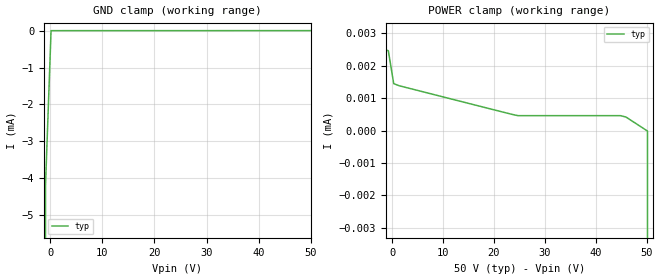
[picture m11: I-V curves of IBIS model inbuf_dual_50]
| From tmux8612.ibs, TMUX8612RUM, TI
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| inbuf_dual_50
[Model]   inbuf_dual_50
Model_type   Input
Vinl = 0.8
Vinh = 1.3
|   typ   min   max
C_comp   1.008417e-12   NA   NA
[Voltage Range]   50   NA   NA
[Temperature Range]   27   NA   NA
[Power Clamp Reference]   50   NA   NA
[GND Clamp Reference]   0   NA   NA
[GND Clamp]
|   Voltage   I(typ)   I(min)   I(max)
-55V      -12.6A     NA         NA
-1.97V    -208.8mA   NA         NA
-909.1mV  -4.166mA   NA         NA
151.5mV   15.32nA    NA         NA
50V       2.185uA    NA         NA
[POWER Clamp]
|   Voltage   I(typ)   I(min)   I(max)
-5V       5.025uA    NA         NA
-3.939V   2.591uA    NA         NA
-757.6mV  2.464uA    NA         NA
303mV     1.446uA    NA         NA
1.364V    1.383uA    NA         NA
24.7V     459.2nA    NA         NA
44.85V    458.8nA    NA         NA
45.91V    417nA      NA         NA
50.15V    -15.83nA   NA         NA
51.21V    -44.85mA   NA         NA
100V      -11.45A    NA         NA
